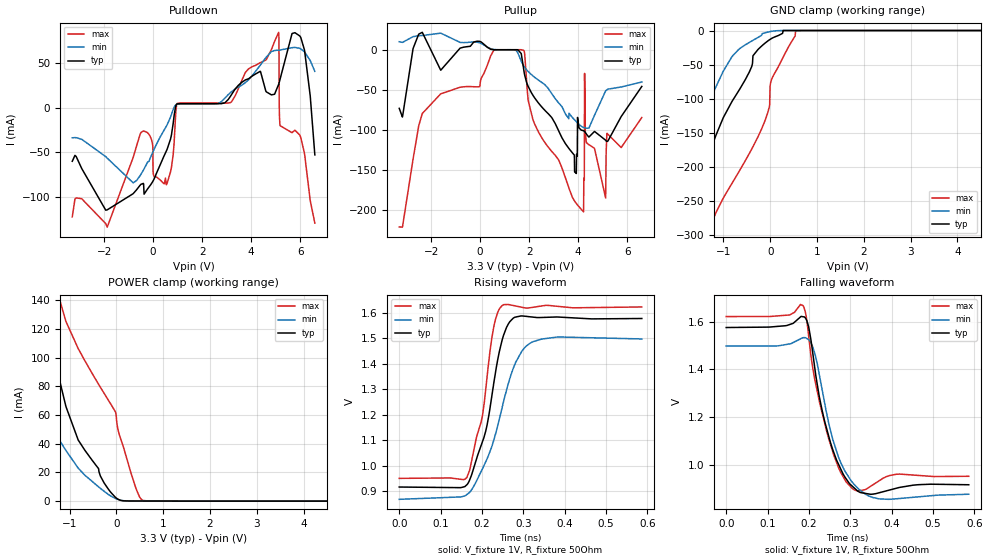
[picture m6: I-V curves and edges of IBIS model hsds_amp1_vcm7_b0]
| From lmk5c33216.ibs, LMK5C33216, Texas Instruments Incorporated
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[Model]   hsds_amp1_vcm7_b0
Model_type   Output
Polarity   Non-Inverting
Vmeas = 1.25
Vref = 1
Cref = 0pF
Rref = 50
|   typ   min   max
C_comp   0.65pF   0.575pF   0.725pF
[Voltage Range]   3.3   3.135   3.465
[Temperature Range]   50   135   -40
[Pullup Reference]   3.3   3.135   3.465
[Pulldown Reference]   -0   0   0
[Power Clamp Reference]   3.3   3.135   3.465
[GND Clamp Reference]   0   0   0
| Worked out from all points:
|   slope of the pulldown table from 0 to 0.495 V, typ, clamps not added: 16.2 ohm
|   slope of the pullup table from 0 to 0.495 V, typ, clamps not added: 50.1 ohm
|   falling waveform, V_fixture 1V, R_fixture 50Ohm: 20-80 % time 49.5ps typ, 53.6ps min, 49.2ps max; typ from 1.58 V to 0.915 V
|   rising waveform, V_fixture 1V, R_fixture 50Ohm: 20-80 % time 50.4ps typ, 70.3ps min, 39.4ps max; typ from 0.917 V to 1.58 V
[Pulldown]
|   Voltage   I(typ)   I(min)   I(max)
-3.3V     -59.78mA   -33.69mA   -121.6mA
-1.874V   -113.9mA   -56.29mA   -133.1mA
-815.1mV  -95.86mA   -83.79mA   -55.54mA
-231mV    -90.74mA   -60.99mA   -28.05mA
541.2mV   -48.26mA   -20.69mA   -85.86mA
957mV     3.583mA    3.534mA    2.974mA
3.165V    12.92mA    16.83mA    5.657mA
5.125V    25.95mA    63.88mA    83.72mA
5.155V    28.78mA    63.96mA    -9.059mA
5.184V    31.93mA    64.06mA    -20.2mA
6.026V    78.04mA    65.34mA    -33.34mA
6.6V      -52.67mA   40.27mA    -128.6mA
[GND Clamp]
|   Voltage   I(typ)   I(min)   I(max)
-3.3V     -892.9mA   -765.6mA   -1.068A
-1.924V   -314.6mA   -288.5mA   -459.9mA
-1.815V   -287mA     -251.4mA   -425.6mA
-1.478V   -218.2mA   -143.5mA   -333.1mA
-1.162V   -154.3mA   -82.94mA   -268mA
-815.1mV  -104mA     -38.12mA   -224.4mA
-171.6mV  -22.09mA   -4.573mA   -142.5mA
-13.2mV   -13.46mA   -1.685mA   -109.6mA
-3.3mV    -13.01mA   -1.546mA   -81.32mA
26.4mV    -11.77mA   -1.169mA   -72.35mA
551.1mV   0A         -83.65nA   -744uA
6.6V      0A         0A         0A
[Pullup]
|   Voltage   I(typ)   I(min)   I(max)
-3.3V     -72.99mA   9.919mA    -220.5mA
-2.36V    21.64mA    17.65mA    -79.41mA
570.9mV   -1.131uA   198.8uA    -437.5uA
1.789V    -26.23mA   -20.59mA   -1.255mA
3.858V    -152.2mA   -87.32mA   -188.5mA
4.224V    -100.9mA   -96.71mA   -201.8mA
4.254V    -101.5mA   -97mA      -162mA
4.264V    -101.8mA   -97.09mA   -29.49mA
4.333V    -104.7mA   -97.63mA   -114.6mA
5.125V    -112.7mA   -51.16mA   -184.6mA
5.174V    -114.2mA   -49.98mA   -104.4mA
6.6V      -45.69mA   -40.22mA   -84.42mA
[POWER Clamp]
|   Voltage   I(typ)   I(min)   I(max)
-3.3V     330.7mA    180mA      566.4mA
-2.736V   200mA      135.8mA    401.6mA
-1.647V   138.3mA    65.17mA    197.7mA
-1.459V   117.6mA    55.06mA    168.7mA
-1.082V   66.76mA    35.64mA    126mA
-815.1mV  42.67mA    23.06mA    106.5mA
-3.3mV    2.23mA     1.644mA    59.85mA
46.2mV    1.16mA     1.045mA    48.48mA
313.5mV   86.42uA    94.45uA    19.62mA
491.7mV   74.41uA    72.76uA    3.272mA
570.9mV   69.96uA    68.47uA    464.3uA
6.6V      0A         0A         0A
[Ramp]
R_load = 50
|   typ   min   max
dV/dt_r   0.395942/5.05438e-11   0.376782/7.03406e-11   0.402743/3.96361e-11
dV/dt_f   0.396455/4.95306e-11   0.373617/5.33284e-11   0.402743/4.91154e-11
[Falling Waveform]
V_fixture = 1V
V_fixture_min = 0.95V
V_fixture_max = 1.05V
R_fixture = 50Ohm
C_fixture = 0F
|   Time   V(typ)   V(min)   V(max)
0s        1.576V     1.498V     1.622V
151.4ps   1.587V     1.506V     1.628V
186ps     1.621V     1.533V     1.668V
198.9ps   1.581V     1.525V     1.546V
214.3ps   1.403V     1.466V     1.356V
242.7ps   1.151V     1.216V     1.141V
271.1ps   1.003V     1.033V     989.3mV
305.2ps   908.3mV    924.8mV    898.6mV
368.5ps   880.9mV    855.9mV    930.5mV
586.3ps   915.1mV    875.3mV    950.6mV
[Rising Waveform]
V_fixture = 1V
V_fixture_min = 0.95V
V_fixture_max = 1.05V
R_fixture = 50Ohm
C_fixture = 0F
|   Time   V(typ)   V(min)   V(max)
0s        916.8mV    868.6mV    950.6mV
163.3ps   925.6mV    887.2mV    953.7mV
200.6ps   1.092V     986.4mV    1.191V
208.9ps   1.135V     1.015V     1.296V
227.8ps   1.316V     1.096V     1.538V
248.2ps   1.489V     1.225V     1.627V
263.2ps   1.554V     1.319V     1.631V
281.5ps   1.582V     1.405V     1.626V
321.4ps   1.582V     1.484V     1.62V
586.3ps   1.577V     1.497V     1.622V
